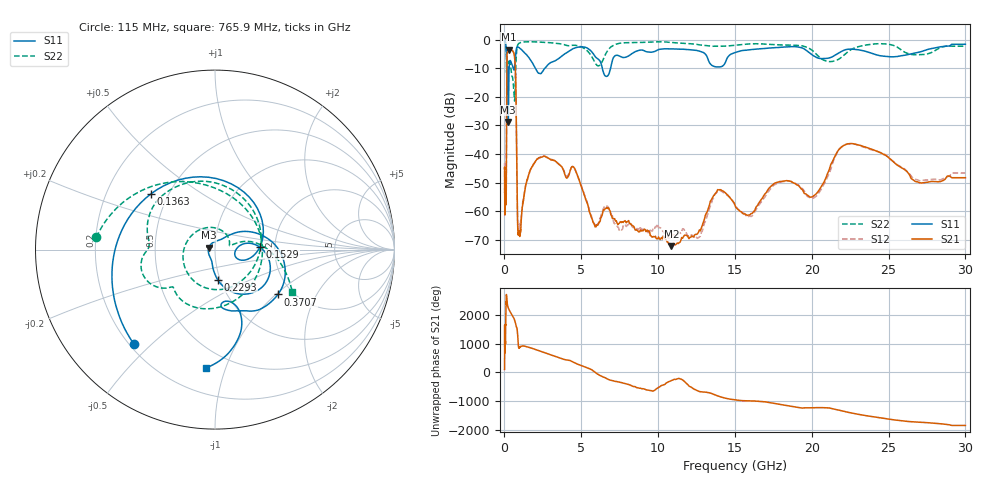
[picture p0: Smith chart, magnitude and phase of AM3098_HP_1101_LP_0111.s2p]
! Date/Time: Thu, Feb 28, 2019 8:45 AM
! Network Analyzer: Agilent Technologies E8364B Rev: A.07.50.67
! Sweep from 0.010 to 30.000 GHz, 1601 Points, Sweep Type: LOG
! Power Supply: 5.022 V, 0.002 A
# Hz S DB R 50
!freq MagS11 AngS11 MagS21 AngS21 MagS12 AngS12 MagS22 AngS22
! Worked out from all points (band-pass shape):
!   1601 points, 10 MHz to 30 GHz, reference 50 ohm
!   highest |S21| = -3.47 dB at 266.5 MHz (marker M1); lowest = -72.3 dB at 10.86 GHz (marker M2)
!   |S21| within 3 dB of the highest: 158.6 MHz to 665.6 MHz (506.9 MHz wide, 123 % of centre)
!   lowest |S11| = -28.8 dB at 249.7 MHz (marker M3), VSWR 1.08, Z = 46.6 + j0.991 ohm
!   |S11| at or under -10 dB: 207.6 MHz to 302.8 MHz (95.19 MHz wide, 37.3 % of centre); 2.009 GHz to 2.642 GHz (633.6 MHz wide, 27.2 % of centre); 6.369 GHz to 6.906 GHz (537.6 MHz wide, 8.1 % of centre)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
!   |S22| runs from -21.5 to -0.5 dB; largest |S21 - S12| = 0.012
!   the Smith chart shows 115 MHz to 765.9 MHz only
!   S11 on the Smith chart (normalised r, x): 115 MHz: 0.22, -0.44; 136.3 MHz: 0.40, +0.32; 152.9 MHz: 1.67, +0.06; 229.3 MHz: 0.97, -0.34; 370.7 MHz: 1.68, -1.03; 765.9 MHz: 0.37, -0.86
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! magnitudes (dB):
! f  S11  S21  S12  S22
! 10 MHz  -0.4  -45.3  -43.2  -0.5
! 38.04 MHz  -0.3  -57.8  -56.6  -0.8
! 115 MHz  -3.2  -54.6  -54.1  -3.5
! 136.3 MHz  -6.5  -25.9  -25.8  -10.9
! 144.7 MHz  -8.7  -14.3  -14.2  -10.7
! 152.9 MHz  -12.0  -8.3  -8.3  -9.4
! 229.3 MHz  -15.5  -3.7  -3.7  -8.3
! 249.7 MHz  -28.8  -3.5  -3.5  -8.7
! 266.5 MHz  -18.8  -3.5  -3.4  -8.6
! 370.7 MHz  -7.3  -3.7  -3.7  -8.1
! 550.5 MHz  -9.6  -4.1  -4.1  -14.0
! 692.9 MHz  -7.5  -8.5  -8.4  -17.8
! 765.9 MHz  -3.6  -25.5  -25.4  -6.2
! 898.9 MHz  -2.6  -68.2  -65.3  -1.5
! 2.084 GHz  -10.8  -42.0  -42.3  -0.8
! 4.503 GHz  -3.1  -44.6  -44.8  -2.0
! 5.87 GHz  -5.7  -65.0  -64.6  -7.8
! 7.926 GHz  -6.1  -64.1  -65.4  -1.1
! 10.86 GHz  -3.2  -72.3  -69.6  -1.0
! 20.1 GHz  -5.6  -54.8  -55.5  -4.1
! 22.56 GHz  -3.3  -36.4  -36.5  -3.5
! 30 GHz  -1.6  -48.3  -46.7  -2.3
